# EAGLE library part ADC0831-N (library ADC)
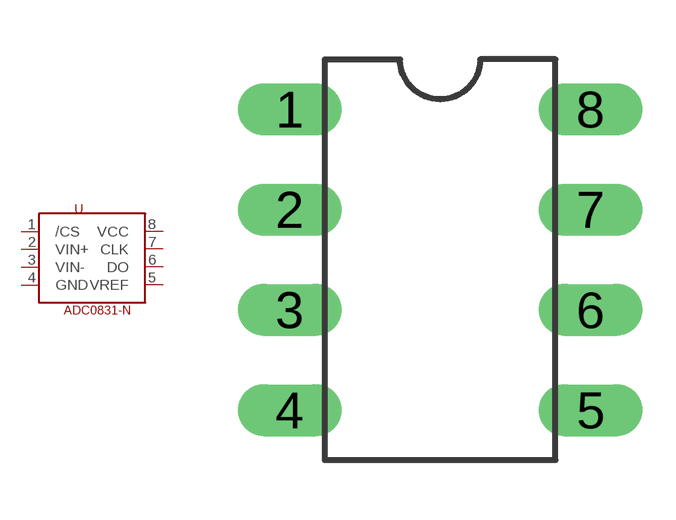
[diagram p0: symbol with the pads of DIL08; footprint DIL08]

Designator prefix -

## ADC0831-N  [DIL08]
1  /CS
2  VIN+
3  VIN-
4  GND
5  VREF
6  DO
7  CLK
8  VCC

## Footprint DIL08 (pad centres in mm)
drill 0.813 long: 1 -3.81,3.81; 2 -3.81,1.27; 3 -3.81,-1.27; 4 -3.81,-3.81; 5 3.81,-3.81; 6 3.81,-1.27; 7 3.81,1.27; 8 3.81,3.81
